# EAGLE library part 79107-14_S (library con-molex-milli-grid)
RECEPTACAL
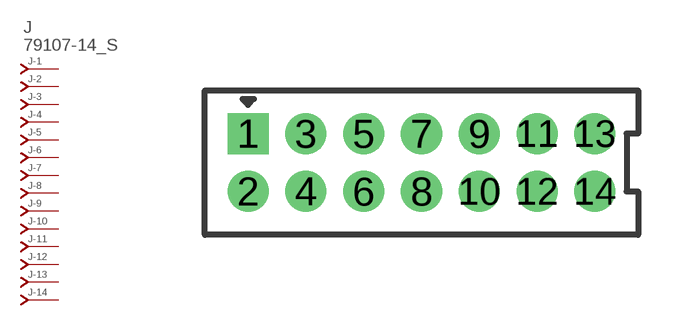
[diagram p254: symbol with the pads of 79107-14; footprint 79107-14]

Designator prefix J; gates -1=J-NV -2=J-N -3=J-N -4=J-N -5=J-N -6=J-N -7=J-N -8=J-N -9=J-N -10=J-N -11=J-N -12=J-N -13=J-N -14=J-N

## 79107-14_S  [79107-14]
1  -1:J  pas
2  -2:J  pas
3  -3:J  pas
4  -4:J  pas
5  -5:J  pas
6  -6:J  pas
7  -7:J  pas
8  -8:J  pas
9  -9:J  pas
10  -10:J  pas
11  -11:J  pas
12  -12:J  pas
13  -13:J  pas
14  -14:J  pas

## Footprint 79107-14 (pad centres in mm)
RECEPTACAL Dual Row, Vertical, Through-Hole
drill 0.914 square: 1 -6,1
drill 0.914: 2 -6,-1; 3 -4,1; 4 -4,-1; 5 -2,1; 6 -2,-1; 7 0,1; 8 0,-1; 9 2,1; 10 2,-1; 11 4,1; 12 4,-1; 13 6,1; 14 6,-1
